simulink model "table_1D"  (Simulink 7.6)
settings: Solver=ode15s  StartTime=0.0  StopTime=10.0  RelTol=1e-3
libraries: fl_lib x2, nesl_utility x2

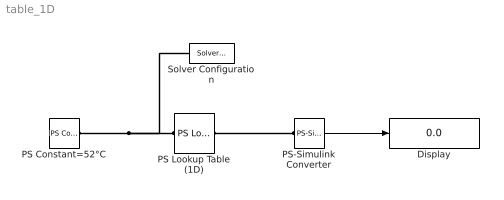
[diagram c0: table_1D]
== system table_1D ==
  Display : Display
  PS Constant=52°C : fl_lib/Physical Signals/Sources/PS Constant  DialogController=NetworkEngine.DynNeDlgSource  SystemSampleTime=-1  constant=52  LocalVarLogging=[]
  PS Lookup Table (1D) : fl_lib/Physical Signals/Lookup Tables/PS Lookup Table (1D)  DialogController=NetworkEngine.DynNeDlgSource  SystemSampleTime=-1  x_t="[0     5    10    15    20    25    30    35    40    45    50  55    60    65    70    75    80    85    90    95   100]"  y_t="[46.2993   46.3111   46.3228   46.3346   46.3463   46.3581  46.3698   46.3816   46.3933 46.4051   46.4168   46.4286  46.4403   46.4521   46.4638   46.4756   46.4873   46.4991 46.5108   46.5226   46.5343]"  interp_method=1  extrap_method=1  dbg=0  LocalVarLogging=[]
  PS-Simulink Converter : nesl_utility/PS-Simulink Converter  DialogController=NetworkEngine.DynNeUtilDlgSource  SystemSampleTime=-1  PhysicalDomain=network_engine_domain  LeftPortType=input  RightPortType=output  SubClassName=ps_output  Unit=1  AffineConversion=off
  Solver Configuration : nesl_utility/Solver Configuration  DialogController=NetworkEngine.DynNeUtilDlgSource  SystemSampleTime=-1  PhysicalDomain=network_engine_domain  LeftPortType=input  RightPortType=generic  SubClassName=solver  Accelerate=off  Profile=off  ResidualTolerance=1e-9  MaxNonlinIter=12  MaxModeIter=2  DoFixedCost=off  UseLocalSampling=off  DoDC=off  LinearAlgebra=Sparse  LocalSolverSampleTime=.001  LocalSolverChoice=NE_BACKWARD_EULER_ADVANCER  UseLocalSolver=off
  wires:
  PS-Simulink Converter/1 -> Display/1
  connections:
  PS Constant=52°C/RConn1 -- PS Lookup Table (1D)/LConn1 -- Solver Configuration/RConn1
  PS Lookup Table (1D)/RConn1 -- PS-Simulink Converter/LConn1
